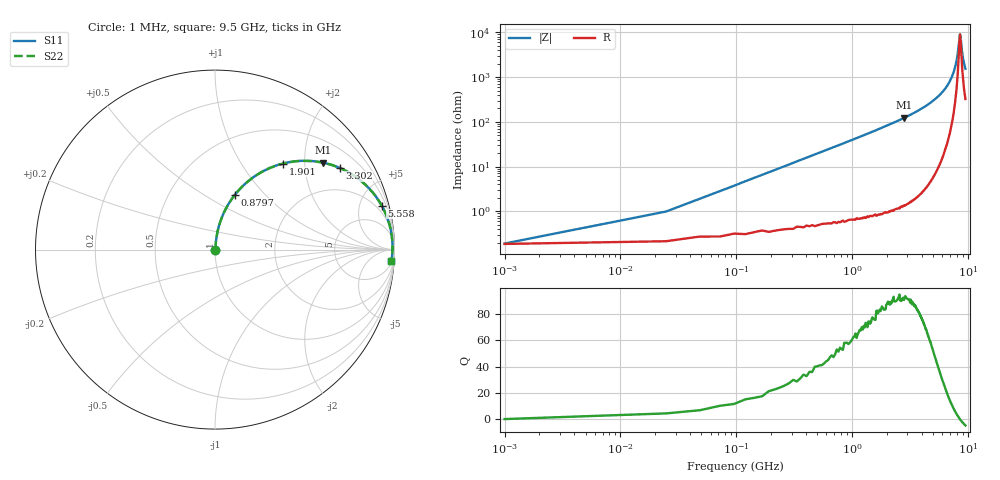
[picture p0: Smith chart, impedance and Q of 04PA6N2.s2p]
! Coilcraft 0402PA-6N2 Chip Inductor
! 11 March 2004
# MHZ S MA R 50
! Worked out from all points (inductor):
!   401 points, 1 MHz to 9.5 GHz, reference 50 ohm
!   read as one part in series: L = 6.18 nH near 48.49 MHz
!   highest Q = 92.4 at 2.827 GHz (marker M1), where L = 6.97 nH
!   self-resonance near 8.526 GHz
!   S11 on the Smith chart (normalised r, x): 1 MHz: 1.00, +0.00; 879.7 MHz: 1.01, +0.69; 1.901 GHz: 1.02, +1.56; 3.302 GHz: 1.03, +3.02; 5.558 GHz: 1.20, +7.50; 9.5 GHz: 7, -30
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1  0.001761 12.7  0.998 -0.0  0.998 -0.0  0.001761 12.7
72.242  0.028 82.6  0.997 -1.6  0.997 -1.6  0.028 82.6
119.738  0.047 83.4  0.996 -2.7  0.996 -2.7  0.047 83.4
190.98  0.074 82.9  0.994 -4.2  0.994 -4.2  0.074 82.9
309.717  0.12 81.1  0.989 -6.9  0.989 -6.9  0.12 81.1
452.202  0.173 78.5  0.98 -10.0  0.98 -10.0  0.173 78.5
879.657  0.326 70.0  0.94 -19.0  0.94 -19.0  0.326 70.0
1592.082  0.537 56.8  0.836 -32.5  0.836 -32.5  0.537 56.8
1900.8  0.611 51.7  0.784 -37.7  0.784 -37.7  0.611 51.7
2826.952  0.774 38.7  0.625 -50.7  0.625 -50.7  0.774 38.7
3183.165  0.817 34.6  0.567 -54.8  0.567 -54.8  0.817 34.6
3301.902  0.83 33.3  0.549 -56.1  0.549 -56.1  0.83 33.3
4750.5  0.932 20.3  0.348 -68.7  0.348 -68.7  0.932 20.3
5557.915  0.96 14.8  0.256 -73.7  0.256 -73.7  0.96 14.8
6341.583  0.977 10.2  0.178 -77.4  0.178 -77.4  0.977 10.2
7243.988  0.986 5.6  0.099 -79.2  0.099 -79.2  0.986 5.6
7932.665  0.989 2.5  0.045 -74.6  0.045 -74.6  0.989 2.5
8217.635  0.989 1.3  0.026 -64.1  0.026 -64.1  0.989 1.3
8478.858  0.989 0.3  0.012 -22.5  0.012 -22.5  0.989 0.3
8550.1  0.989 -0.0  0.011 1.3  0.011 1.3  0.989 -0.0
9025.05  0.987 -1.9  0.035 67.2  0.035 67.2  0.987 -1.9
9500  0.985 -3.6  0.064 74.3  0.064 74.3  0.985 -3.6
